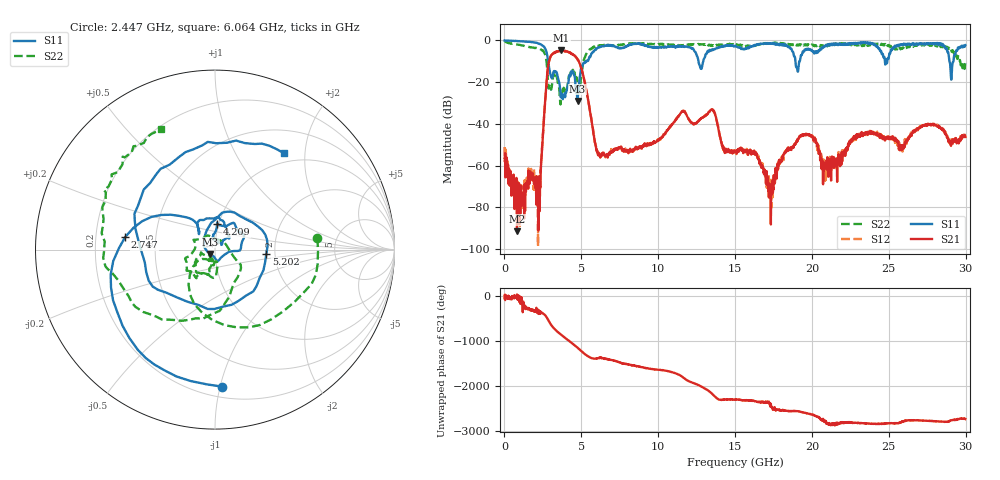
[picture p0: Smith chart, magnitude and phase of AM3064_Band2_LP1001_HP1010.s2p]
# Hz S DB R 50.0
!freq dBS11 angS11 dBS21 angS21 dBS12 angS12 dBS22 angS22
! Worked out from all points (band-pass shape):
!   1600 points, 10 MHz to 29.98 GHz, reference 50 ohm
!   highest |S21| = -4.83 dB at 3.703 GHz (marker M1); lowest = -91.5 dB at 816 MHz (marker M2)
!   |S21| within 3 dB of the highest: 2.99 GHz to 4.633 GHz (1.643 GHz wide, 43.1 % of centre)
!   lowest |S11| = -29.0 dB at 4.752 GHz (marker M3), VSWR 1.07, Z = 47.4 - j2.3 ohm
!   |S11| at or under -10 dB: 2.839 GHz to 5.338 GHz (2.499 GHz wide, 61.1 % of centre); 12.62 GHz to 12.93 GHz (313.8 MHz wide, 2.46 % of centre); 28.94 GHz to 29.2 GHz (257.7 MHz wide, 0.886 % of centre)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
!   |S22| runs from -30.7 to -0.3 dB; largest |S21 - S12| = 0.02
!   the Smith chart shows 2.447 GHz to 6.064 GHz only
!   S11 on the Smith chart (normalised r, x): 2.447 GHz: 0.28, -1.01; 2.747 GHz: 0.33, +0.06; 4.209 GHz: 0.98, +0.28; 5.202 GHz: 1.80, -0.09; 6.064 GHz: 0.85, +1.62
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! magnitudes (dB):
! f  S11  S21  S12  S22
! 10 MHz  0.0  -56.4  -51.1  -0.3
! 816 MHz  -0.3  -91.5  -69.1  -1.9
! 2.166 GHz  -1.4  -69.9  -73.6  -3.8
! 2.447 GHz  -2.3  -51.0  -51.1  -4.8
! 2.747 GHz  -5.9  -19.1  -19.1  -10.9
! 3.703 GHz  -25.3  -4.8  -5.0  -24.9
! 4.209 GHz  -16.9  -5.7  -5.7  -16.9
! 4.752 GHz  -29.0  -8.9  -8.9  -20.9
! 5.015 GHz  -12.9  -13.8  -13.7  -15.0
! 5.202 GHz  -10.8  -19.3  -19.3  -8.6
! 6.064 GHz  -3.6  -53.7  -54.0  -2.6
! 10 GHz  -3.4  -47.6  -47.9  -1.8
! 13.51 GHz  -4.5  -33.1  -33.0  -2.4
! 15 GHz  -2.6  -53.2  -54.2  -1.8
! 16.3 GHz  -2.1  -54.8  -54.2  -2.2
! 17.35 GHz  -1.3  -69.0  -73.3  -1.2
! 18.27 GHz  -2.5  -53.5  -53.4  -1.8
! 19.99 GHz  -4.6  -45.7  -46.2  -2.0
! 20.97 GHz  -2.6  -57.2  -63.1  -2.4
! 25 GHz  -8.2  -46.0  -46.7  -2.2
! 29.08 GHz  -17.5  -48.3  -47.6  -5.2
! 29.98 GHz  -2.3  -46.3  -45.8  -10.9
